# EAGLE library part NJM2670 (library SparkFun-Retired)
Dual H-bridge driver
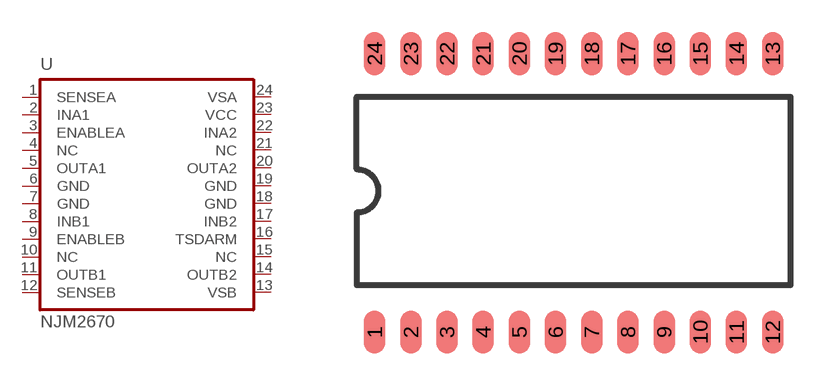
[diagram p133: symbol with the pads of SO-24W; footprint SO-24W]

Designator prefix -

## NJM2670SMD  [SO-24W]
1  SENSEA
2  INA1
3  ENABLEA
4  NC  in
5  OUTA1  pwr
6  GND  pwr
7  GND
8  INB1
9  ENABLEB
10  NC
11  OUTB1
12  SENSEB
13  VSB
14  OUTB2
15  NC
16  TSDARM
17  INB2
18  GND
19  GND  pwr
20  OUTA2  pwr
21  NC
22  INA2
23  VCC
24  VSA

## Footprint SO-24W (pad centres in mm)
smd 0.762 x 1.524: 1 -6.985,-4.953; 2 -5.715,-4.953; 3 -4.445,-4.953; 4 -3.175,-4.953; 5 -1.905,-4.953; 6 -0.635,-4.953; 7 0.635,-4.953; 8 1.905,-4.953; 9 3.175,-4.953; 10 4.445,-4.953; 11 5.715,-4.953; 12 6.985,-4.953; 13 6.985,4.826; 14 5.715,4.826; 15 4.445,4.826; 16 3.175,4.826; 17 1.905,4.826; 18 0.635,4.826; 19 -0.635,4.826; 20 -1.905,4.826; 21 -3.175,4.826; 22 -4.445,4.826; 23 -5.715,4.826; 24 -6.985,4.826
